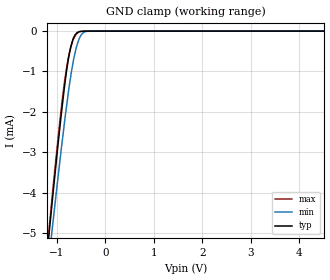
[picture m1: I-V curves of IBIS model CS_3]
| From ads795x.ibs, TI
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|   Input CS model 3V
[Model]   CS_3
Model_type   Input
|Signals   CS
Vinl = 0.4
Vinh = 2.31
|   typ   min   max
C_comp   6.5646992e-13  7.4011158e-13   5.7746441e-13
[Voltage Range]   3.3   3   3.6
[Temperature Range]   27   125   -40
[Pullup Reference]   3.3   3   3.6
[Pulldown Reference]   0   0   0
[Power Clamp Reference]   3.3   3   3.6
[GND Clamp Reference]   0   0   0
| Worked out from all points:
|   GND clamp passes 1 mA (typ) near -0.80 V on its own axis
[GND Clamp]
|   Voltage   I(typ)   I(min)   I(max)
-3.3V     -32.68mA   -30.38mA   -35.68mA
-1.165V   -5.056mA   -5.66mA    -4.938mA
-1.091V   -4.159mA   -4.847mA   -4.012mA
-976.6mV  -2.806mA   -3.619mA   -2.646mA
-839.9mV  -1.34mA    -2.227mA   -1.217mA
-760.4mV  -666.7uA   -1.488mA   -647.9uA
-717.3mV  -405.7uA   -1.135mA   -417.9uA
-659.7mV  -174.4uA   -727.2uA   -202.3uA
-577.4mV  -33.5uA    -316.7uA   -47.64uA
-458.6mV  -3.039uA   -38.93uA   -3.104uA
-322.1mV  -885.5nA   -969.9nA   -995.7nA
6.59V     0A         0A         0A
[POWER Clamp]
|   No ESD cells to VDD
|   Voltage   I(typ)   I(min)   I(max)
-3.3V     0A         0A         0A
0V        0A         0A         0A
6.6V      0A         0A         0A
